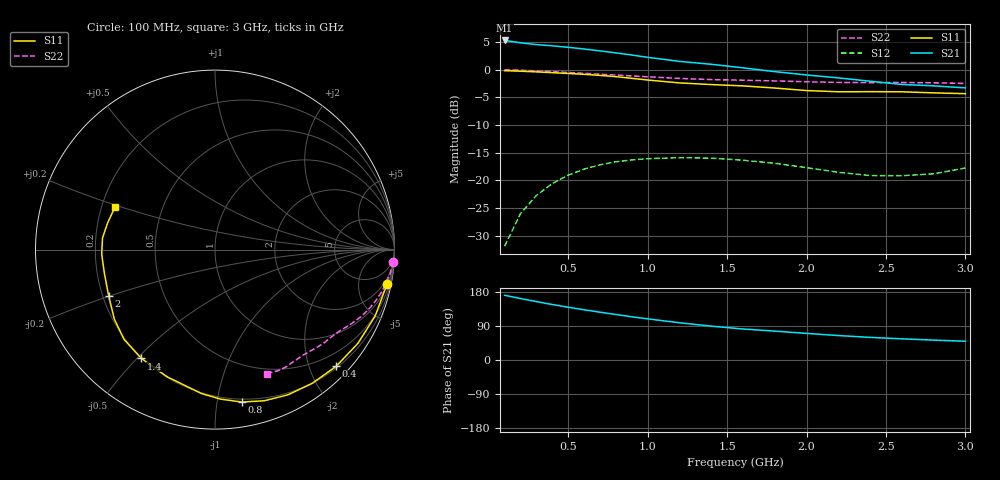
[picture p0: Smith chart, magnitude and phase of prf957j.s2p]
! Filename:  PRF957J.S2P  Version:  3.0
! Philips part #:  PRF957  Date:  Nov 1998
! Bias condition:  Vce=6V, Ic=0.5mA
#  MHz  S  MA  R 50
! Freq  S11  S21  S12  S22
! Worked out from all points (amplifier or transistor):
!   20 points, 100 MHz to 3 GHz, reference 50 ohm
!   highest |S21| = 5.2 dB at 100 MHz (marker M1)
!   |S21| within 3 dB of that: start of sweep to 990.2 MHz
!   unconditionally stable (mu >= 1): 2.297 GHz to end of sweep
!   at 400 MHz: K = 0.12, MSG = 12.4 dB, |S12| = -20.6 dB
!   at 1.2 GHz: K = 0.38, MSG = 8.7 dB, |S12| = -15.9 dB
!   at 3 GHz: K = 1.25, MAG = 4.2 dB, |S12| = -17.7 dB
!   lowest NFmin = 0.96 dB at 500 MHz
!   S11 on the Smith chart (normalised r, x): 100 MHz: 1.16, -9.92; 400 MHz: 0.23, -2.46; 800 MHz: 0.18, -1.17; 1.4 GHz: 0.20, -0.51; 2 GHz: 0.22, -0.20; 3 GHz: 0.26, +0.19
100  0.9772 -11.4  1.829 170.8  0.02558 82.8  0.9957 -3.9
200  0.9663 -22.4  1.742 162.2  0.05026 76.4  0.9854 -7.6
300  0.9524 -33.3  1.678 154.1  0.07326 70.3  0.972 -11.1
400  0.9371 -43.9  1.637 146.4  0.09381 64.5  0.9573 -14.4
500  0.9213 -53.9  1.587 139.2  0.1116 59.5  0.9404 -17.6
600  0.9054 -63.3  1.531 132.6  0.1266 54.8  0.9237 -20.4
700  0.8858 -72.0  1.473 126.2  0.1385 50.5  0.9076 -22.9
800  0.8621 -80.1  1.413 120.1  0.1474 46.4  0.892 -25.1
900  0.8335 -87.9  1.352 114.0  0.1532 42.8  0.8758 -27.1
1000  0.805 -95.5  1.289 108.6  0.1571 39.6  0.8604 -29.1
1200  0.7577 -110.4  1.185 98.4  0.1606 34.1  0.8316 -32.8
1400  0.732 -124.1  1.115 89.4  0.159 29.8  0.8121 -36.5
1600  0.7121 -135.4  1.036 81.8  0.1522 27.8  0.801 -40.0
1800  0.6811 -145.5  0.9575 76.2  0.1429 28.0  0.7894 -43.2
2000  0.6465 -156.3  0.8941 70.2  0.1305 29.6  0.7762 -46.6
2200  0.6304 -167.7  0.8407 64.6  0.1185 33.9  0.7652 -50.6
2400  0.6318 -177.6  0.785 59.6  0.1108 41.8  0.762 -55.0
2600  0.6302 174.2  0.7338 55.9  0.1103 52.9  0.764 -59.1
2800  0.6164 166.0  0.713 52.5  0.1148 65.1  0.7594 -62.9
3000  0.6058 156.8  0.6833 49.5  0.1296 75.8  0.7489 -67.3
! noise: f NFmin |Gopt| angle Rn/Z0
500  0.96  0.75  37  0.72
800  1.21  0.72  57  0.66
900  1.44  0.63  63  0.62
1000  1.83  0.61  69  0.62
1500  1.84  0.61  111  0.39
2000  2.43  0.59  162  0.11
